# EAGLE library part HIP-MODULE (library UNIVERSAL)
HIP MINI MODULE
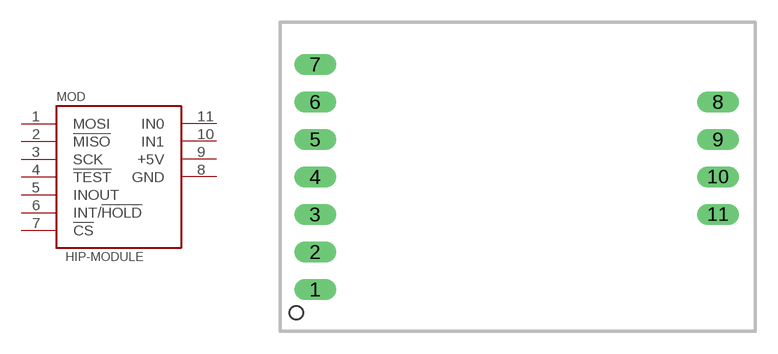
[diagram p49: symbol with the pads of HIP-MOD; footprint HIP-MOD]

Designator prefix MOD

## HIP-MODULE  [HIP-MOD]
1  MOSI
2  !MISO
3  SCK
4  !TEST
5  INOUT
6  INT/!HOLD
7  !CS
8  GND
9  +5V
10  IN1
11  IN0

## Footprint HIP-MOD (pad centres in mm)
drill 0.8 pad 1.422 long: 1 2.223,2.54; 2 2.223,5.08; 3 2.223,7.62; 4 2.223,10.16; 5 2.223,12.7; 6 2.223,15.24; 7 2.223,17.78; 8 29.527,15.24; 9 29.527,12.7; 10 29.527,10.16; 11 29.527,7.62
